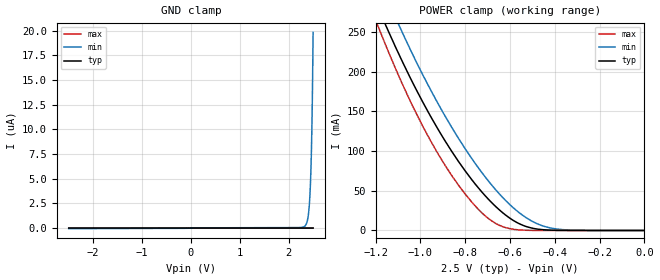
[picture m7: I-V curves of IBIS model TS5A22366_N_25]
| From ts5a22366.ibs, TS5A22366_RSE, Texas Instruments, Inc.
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[Model]   TS5A22366_N_25
Model_type  Terminator
| variable   typ   min   max
C_comp   39.34pF   36.96pF   42.40pF
| C_tri-state   39.34pF   36.96pF   42.40pF
[Temperature Range]   40   100   -40
| Ambient temperature   25   85   -40
[Voltage range]   2.5   2.3   2.7
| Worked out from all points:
|   POWER clamp passes 1 mA (typ) near -0.45 V on its own axis
[GND Clamp]
| TS5A22366_N_25
|   Voltage   I(typ)   I(min)   I(max)
-2.5V     -657.8pA   -62.36nA   -148.3pA
2.325V    356.3pA    168.9nA    22.15pA
2.365V    362.9pA    462.8nA    23.31pA
2.395V    371.2pA    1.068uA    24.17pA
2.42V     385pA      2.172uA    24.88pA
2.44V     407.9pA    3.822uA    25.45pA
2.45V     427.2pA    5.058uA    25.73pA
2.46V     455pA      6.681uA    26.02pA
2.475V    522.6pA    10.1uA     26.44pA
2.485V    594.8pA    13.25uA    26.73pA
2.49V     642.8pA    15.17uA    26.87pA
2.5V      771.5pA    19.83uA    27.15pA
[POWER Clamp]
| TS5A22366_N_25
|   Voltage   I(typ)   I(min)   I(max)
-2.5V     1.623A     1.654A     1.77A
-1.19V    281.5mA    319.9mA    258.1mA
-1.175V   271.6mA    309.8mA    247.4mA
-1.14V    249.1mA    286.7mA    223.2mA
-1.08V    212.4mA    248.9mA    184.1mA
-925mV    129.3mA    161.7mA    98.37mA
-800mV    75mA       102.9mA    45.89mA
-690mV    37.49mA    60.1mA     13.72mA
-570mV    10.16mA    24.91mA    992.2uA
-490mV    2.304mA    9.997mA    78.57uA
-395mV    222.7uA    1.968mA    2.186uA
0V        0A         0A         0A
